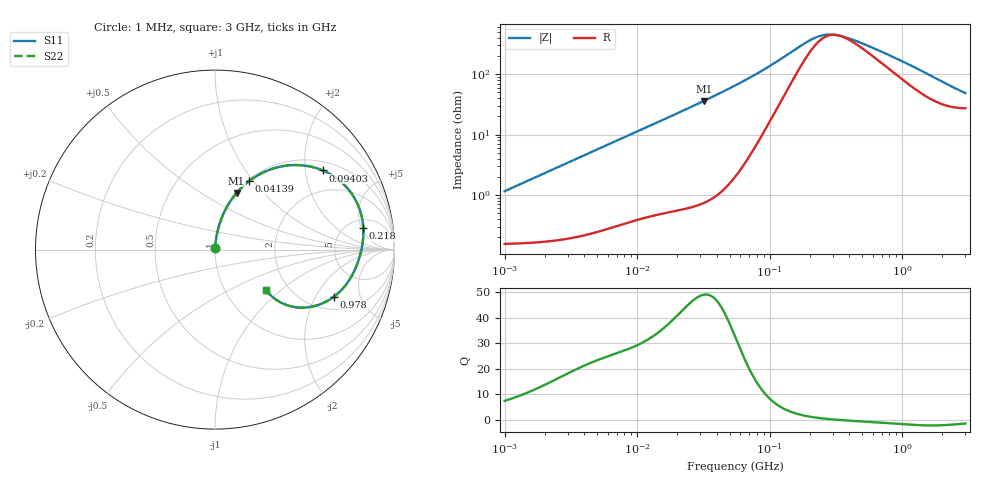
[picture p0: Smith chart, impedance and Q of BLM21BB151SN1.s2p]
! BLM21BB151SN1
# Hz S RI R 50
!Freq.(Hz) S11(Real) S11(Imag) S21(Real) S21(Imag) S12(Real) S12(Imag) S22(Real) S22(Imag)
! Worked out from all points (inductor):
!   401 points, 1 MHz to 3 GHz, reference 50 ohm
!   read as one part in series: L = 182 nH near 1.041 MHz
!   highest Q = 48.9 at 31.9 MHz (marker M1), where L = 180 nH
!   self-resonance near 321.7 MHz
!   S11 on the Smith chart (normalised r, x): 1 MHz: 1.00, +0.02; 41.39 MHz: 1.02, +0.95; 94.03 MHz: 1.26, +2.49; 218 MHz: 6.85, +5.36; 978 MHz: 2.71, -2.88; 3 GHz: 1.54, -0.81
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1000000  0.00167 0.0114  0.9983 -0.0114  0.9983 -0.0114  0.00167 0.0114
3823119  0.00397 0.0433  0.996 -0.0433  0.996 -0.0433  0.00397 0.0433
8017732  0.0114 0.0891  0.9886 -0.0891  0.9886 -0.0891  0.0114 0.0891
1.461624e7  0.0304 0.1578  0.9696 -0.1578  0.9696 -0.1578  0.0304 0.1578
2.270269e7  0.0655 0.2362  0.9345 -0.2362  0.9345 -0.2362  0.0655 0.2362
3.190472e7  0.1201 0.3151  0.8799 -0.3151  0.8799 -0.3151  0.1201 0.3151
4.138676e7  0.1896 0.3812  0.8104 -0.3812  0.8104 -0.3812  0.1896 0.3812
5.477226e7  0.3013 0.4437  0.6987 -0.4437  0.6987 -0.4437  0.3013 0.4437
7.248696e7  0.4505 0.4712  0.5495 -0.4712  0.5495 -0.4712  0.4505 0.4712
9.402997e7  0.601 0.4409  0.399 -0.4409  0.399 -0.4409  0.601 0.4409
1.375402e8  0.7653 0.306  0.2347 -0.306  0.2347 -0.306  0.7653 0.306
2.094008e8  0.8253 0.133  0.1747 -0.133  0.1747 -0.133  0.8253 0.133
2.179536e8  0.8263 0.1186  0.1737 -0.1186  0.1737 -0.1186  0.8263 0.1186
2.716345e8  0.8238 0.0473  0.1762 -0.0473  0.1762 -0.0473  0.8238 0.0473
3.385367e8  0.813 -0.0134  0.187 0.0134  0.187 0.0134  0.813 -0.0134
4.480278e8  0.7919 -0.0821  0.2081 0.0821  0.2081 0.0821  0.7919 -0.0821
8.005644e8  0.7113 -0.2177  0.2887 0.2177  0.2887 0.2177  0.7113 -0.2177
9.779672e8  0.6637 -0.2615  0.3363 0.2615  0.3363 0.2615  0.6637 -0.2615
1.320433e9  0.5665 -0.3113  0.4335 0.3113  0.4335 0.3113  0.5665 -0.3113
1.712864e9  0.4635 -0.3224  0.5365 0.3224  0.5365 0.3224  0.4635 -0.3224
2.359433e9  0.3451 -0.2823  0.6549 0.2823  0.6549 0.2823  0.3451 -0.2823
3e9  0.2857 -0.2264  0.7143 0.2264  0.7143 0.2264  0.2857 -0.2264
